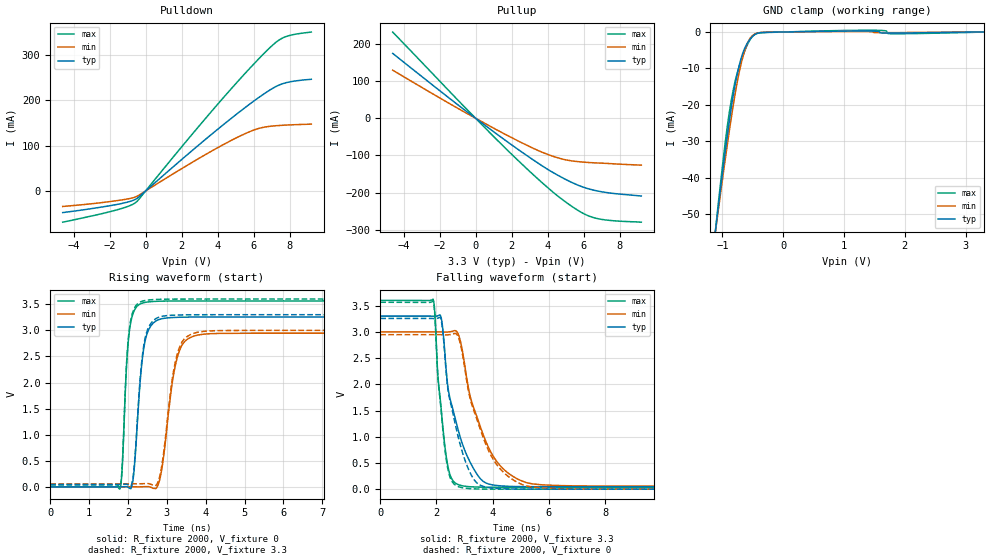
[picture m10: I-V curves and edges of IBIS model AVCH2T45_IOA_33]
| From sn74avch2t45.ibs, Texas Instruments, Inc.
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[Model]   AVCH2T45_IOA_33
Model_type  I/O
Vinl=0.8
Vinh=2.0
Enable   Active-Low
Vref =   0
Rref =   2000
Cref =   15p
Vmeas =   1.65
| variable   typ   min   max
C_comp   4.94pF   3.97pF   5.92pF
| C_pullup   3.99pF   3.01pF   5.23pF
| C_pulldown   4.19pF   3.64pF   4.72pF
| C_tri-state   4.94pF   3.97pF   5.92pF
[Temperature Range]   40   100   -40
| Ambient temperature   25   85   -40
[Voltage range]   3.3   3   3.6
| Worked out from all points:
|   slope of the pulldown table from 0 to 0.495 V, typ, clamps not added: 28.7 ohm
|   slope of the pullup table from 0 to 0.495 V, typ, clamps not added: 27.4 ohm
|   GND clamp passes 1 mA (typ) near -0.49 V on its own axis
|   rising waveform, R_fixture 2000, V_fixture 0: 20-80 % time 204ps typ, 310ps min, 142ps max; typ from 0 V to 3.26 V
|   falling waveform, R_fixture 2000, V_fixture 3.3: 20-80 % time 749ps typ, 1.01ns min, 330ps max; typ from 3.3 V to 0.046 V
|   rising waveform, R_fixture 2000, V_fixture 3.3: 20-80 % time 203ps typ, 308ps min, 142ps max; typ from 0.046 V to 3.3 V
|   falling waveform, R_fixture 2000, V_fixture 0: 20-80 % time 662ps typ, 1.01ns min, 326ps max; typ from 3.26 V to 0 V
[GND Clamp]
| AVCH2T45_IOA_33
|   Voltage   I(typ)   I(min)   I(max)
-4.6V     -599.7mA   -548.3mA   -664.9mA
-1.12V    -55.23mA   -55.37mA   -55.14mA
-1.09V    -51.05mA   -51.59mA   -50.43mA
-920mV    -28.51mA   -30.95mA   -25.9mA
-810mV    -16.17mA   -18.87mA   -14.9mA
-725mV    -9.266mA   -11.11mA   -9.544mA
-630mV    -4.345mA   -4.957mA   -5.066mA
-555mV    -2.184mA   -2.008mA   -2.394mA
-460mV    -638.5uA   -501uA     -616.7uA
1.285V    253.4uA    145.8uA    464.3uA
1.78V     -297.7uA   -185uA     -481uA
3.3V      1.647nA    4.601uA    -26.77uA
[Pulldown]
| AVCH2T45_IOA_33
|   Voltage   I(typ)   I(min)   I(max)
-4.6V     -47.48mA   -33.99mA   -68.59mA
-1.68V    -30.25mA   -21.7mA    -42.42mA
-975mV    -24.15mA   -17.32mA   -33.81mA
-545mV    -17.86mA   -12.84mA   -25.24mA
2.545V    87.52mA    61.96mA    122.8mA
4.505V    151.8mA    106mA      213.5mA
5.905V    194.7mA    132.4mA    274.8mA
6.805V    219.6mA    141.6mA    311.5mA
7.315V    231.2mA    143.7mA    329.3mA
7.73V     237.3mA    144.7mA    338.5mA
8.28V     241.7mA    145.7mA    344.4mA
9.2V      245.6mA    146.9mA    349.3mA
[Pullup]
| AVCH2T45_IOA_33
|   Voltage   I(typ)   I(min)   I(max)
-4.6V     174.2mA    129.1mA    231.4mA
-1.105V   40.58mA    29.86mA    54.82mA
1.575V    -56.66mA   -41.45mA   -76.65mA
3.53V     -122.6mA   -88.07mA   -166.1mA
4.725V    -157.4mA   -108.5mA   -215.1mA
5.775V    -181.6mA   -117mA     -250.3mA
6.525V    -192.9mA   -119.7mA   -266.7mA
7.455V    -200.9mA   -121.9mA   -274.6mA
9.2V      -209mA     -126mA     -279.3mA
[Ramp]
| AVCH2T45_IOA_33
| variable   typ   min   max
dV/dt_r   1.98/2.07E-10   1.79/3.16E-10   2.17/1.45E-10
dV/dt_f   1.97/7.49E-10   1.78/1.01E-09   2.15/3.32E-10
R_load = 2000
[Rising Waveform]
| AVCH2T45_IOA_33
R_fixture =   2000
C_fixture =   0
L_fixture =   0
V_fixture =   0
V_fixture_min = 0
V_fixture_max = 0
|   Time   V(typ)   V(min)   V(max)
0s        37.81nV    120nV      1.948nV
1.795ns   -43.77uV   -5.713uV   -34.48mV
2.05ns    -30.27mV   32.52uV    3.06V
2.14ns    192.7mV    34.52uV    3.341V
2.34ns    2.241V     211.5uV    3.515V
2.495ns   2.945V     4.378mV    3.543V
2.825ns   3.214V     161mV      3.559V
3.31ns    3.251V     2.579V     3.563V
3.915ns   3.255V     2.924V     3.564V
34.99ns   3.256V     2.946V     3.564V
[Falling Waveform]
| AVCH2T45_IOA_33
R_fixture =   2000
C_fixture =   0
L_fixture =   0
V_fixture =   3.3
V_fixture_min = 3
V_fixture_max = 3.6
|   Time   V(typ)   V(min)   V(max)
0s        3.3V       3V         3.6V
1.88ns    3.299V     3V         3.62V
2.17ns    3.26V      2.999V     1.51V
2.365ns   2.15V      2.997V     558.1mV
2.725ns   1.225V     3.003V     99.02mV
2.93ns    850.5mV    2.614V     63.58mV
3.225ns   484.9mV    1.716V     45.33mV
3.92ns    89.59mV    721mV      36.89mV
5.4ns     47.01mV    101.4mV    35.99mV
34.99ns   46.09mV    58.43mV    35.95mV
[Rising Waveform]
| AVCH2T45_IOA_33
R_fixture =   2000
C_fixture =   0
L_fixture =   0
V_fixture =   3.3
V_fixture_min = 3
V_fixture_max = 3.6
|   Time   V(typ)   V(min)   V(max)
0s        46.09mV    58.43mV    35.95mV
1.795ns   46.05mV    58.42mV    1.352mV
2.05ns    15.69mV    58.46mV    3.101V
2.14ns    239.8mV    58.46mV    3.382V
2.34ns    2.294V     58.64mV    3.552V
2.495ns   2.994V     62.82mV    3.579V
2.825ns   3.259V     221.8mV    3.595V
3.305ns   3.295V     2.633V     3.599V
3.915ns   3.3V       2.978V     3.6V
34.99ns   3.3V       3V         3.6V
[Falling Waveform]
| AVCH2T45_IOA_33
R_fixture =   2000
C_fixture =   0
L_fixture =   0
V_fixture =   0
V_fixture_min = 0
V_fixture_max = 0
|   Time   V(typ)   V(min)   V(max)
0s        3.256V     2.946V     3.564V
1.88ns    3.254V     2.946V     3.585V
2.17ns    3.216V     2.945V     1.469V
2.365ns   2.111V     2.942V     505.3mV
2.725ns   1.105V     2.949V     61.67mV
2.935ns   679.9mV    2.543V     26.24mV
3.22ns    287.3mV    1.68V      9.202mV
3.92ns    25.64mV    662.9mV    907.3uV
5.385ns   550.7uV    41.67mV    33.41uV
34.99ns   789.6nV    735.8nV    346.3nV
